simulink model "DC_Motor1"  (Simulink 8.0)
settings: Solver=ode3  StartTime=0.0  StopTime=inf  RelTol=1e-3
InitFcn:
  | dt=0.01;
  | Kp=0.5; Kd=0; Ki=0;
libraries: arduinolib x8, simulink x2

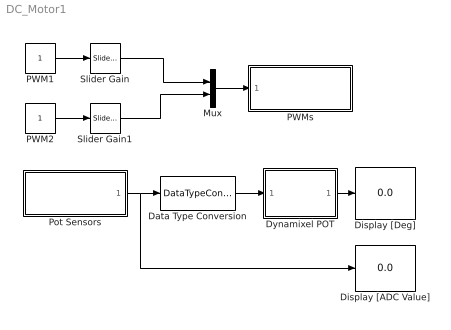
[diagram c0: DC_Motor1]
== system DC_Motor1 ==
  Data Type Conversion : DataTypeConversion  OutDataTypeStr=double
  Display [ADC Value] : Display
  Display [Deg] : Display
  Dynamixel POT : MATLAB Function  TreatAsAtomicUnit=on
  Mux : Mux  Inputs=2
  PWM1 : Constant
  PWM2 : Constant
  PWMs : Subsystem  TreatAsAtomicUnit=on
  Pot Sensors : Subsystem  TreatAsAtomicUnit=on
  Slider Gain : simulink/Math Operations/Slider Gain  low=-255  gain=0  high=255
  Slider Gain1 : simulink/Math Operations/Slider Gain  low=-255  gain=0  high=255
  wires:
  PWM1/1 -> Slider Gain/1
  Mux/1 -> PWMs/1(In1)
  Slider Gain/1 -> Mux/1
  PWM2/1 -> Slider Gain1/1
  Slider Gain1/1 -> Mux/2
  Dynamixel POT/1(y) -> Display [Deg]/1
  Pot Sensors/1(Out1) -> Display [ADC Value]/1, Data Type Conversion/1
  Data Type Conversion/1 -> Dynamixel POT/1(u)

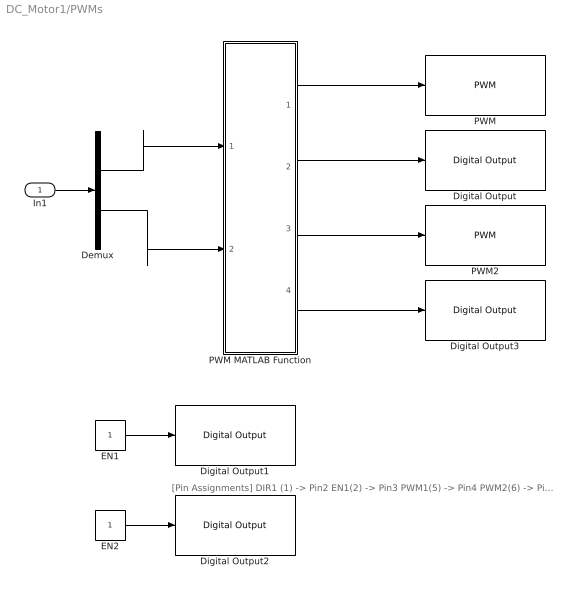
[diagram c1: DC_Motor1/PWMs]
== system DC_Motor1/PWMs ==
  note: [Pin Assignments] DIR1 (1) -> Pin2 EN1(2) -> Pin3 PWM1(5) -> Pin4 PWM2(6) -> Pin5 DIR2 (7) -> Pin6 EN2(8) -> Pin7
  In1 : Inport
  Demux : Demux  Outputs=2
  Digital Output : arduinolib/Digital Output  pinNumber=2
  Digital Output1 : arduinolib/Digital Output  pinNumber=3
  Digital Output2 : arduinolib/Digital Output  pinNumber=7
  Digital Output3 : arduinolib/Digital Output  pinNumber=6
  EN1 : Constant
  EN2 : Constant
  PWM : arduinolib/PWM  pinNumber=4
  PWM MATLAB Function : MATLAB Function  TreatAsAtomicUnit=on
  PWM2 : arduinolib/PWM  pinNumber=5
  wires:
  EN1/1 -> Digital Output1/1
  EN2/1 -> Digital Output2/1
  In1/1 -> Demux/1
  Demux/1 -> PWM MATLAB Function/1(u1)
  Demux/2 -> PWM MATLAB Function/2(u2)
  PWM MATLAB Function/1(pwm1) -> PWM/1
  PWM MATLAB Function/2(dir1) -> Digital Output/1
  PWM MATLAB Function/3(pwm2) -> PWM2/1
  PWM MATLAB Function/4(dir2) -> Digital Output3/1

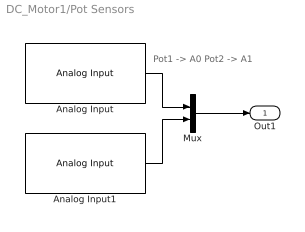
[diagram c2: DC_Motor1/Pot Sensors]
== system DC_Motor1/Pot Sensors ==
  note: Pot1 -> A0 Pot2 -> A1
  Analog Input : arduinolib/Analog Input  pinNumber=0  sampleTime=dt
  Analog Input1 : arduinolib/Analog Input  pinNumber=1  sampleTime=dt
  Mux : Mux  Inputs=2
  Out1 : Outport
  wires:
  Analog Input/1 -> Mux/1
  Analog Input1/1 -> Mux/2
  Mux/1 -> Out1/1

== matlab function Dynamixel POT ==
function y = fcn(u)

MAX_CH=2;
y=zeros(MAX_CH,1);

for ch=1:MAX_CH
    y(ch,1)=(300/1024)*(u(ch,1)-204.8);
end

== matlab function PWMs/PWM
MATLAB Function ==
function [pwm1, dir1, pwm2, dir2] = fcn(u1, u2)

if u1>=0,dir1=1;
else dir1=0; end

if u2>=0,dir2=1;    
else dir2=0; end

pwm1=abs(u1);
pwm2=abs(u2);
% Saturation %
if pwm1>=255, pwm1=255; end
if pwm2>=255, pwm2=255; end
